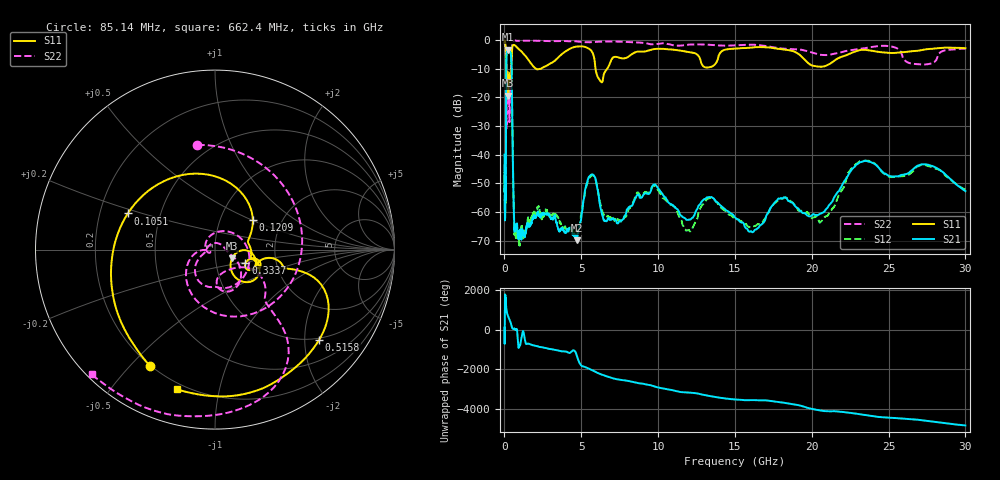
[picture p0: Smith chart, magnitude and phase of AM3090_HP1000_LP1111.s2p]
! Date/Time: Thu, Feb 28, 2019 2:02 PM
! Network Analyzer: Agilent Technologies E8364B Rev: A.07.50.67
! Sweep from 0.010 to 30.000 GHz, 1601 Points, Sweep Type: LOG
! Power Supply: 5.023 V, 0.002 A
# Hz S DB R 50
!freq MagS11 AngS11 MagS21 AngS21 MagS12 AngS12 MagS22 AngS22
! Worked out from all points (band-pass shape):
!   1601 points, 10 MHz to 30 GHz, reference 50 ohm
!   highest |S21| = -3.47 dB at 243.5 MHz (marker M1); lowest = -69.7 dB at 4.71 GHz (marker M2)
!   |S21| within 3 dB of the highest: 124.4 MHz to 442.2 MHz (317.7 MHz wide, 112 % of centre)
!   lowest |S11| = -19.5 dB at 243.5 MHz (marker M3), VSWR 1.24, Z = 60.2 - j5.77 ohm
!   |S11| at or under -10 dB: 118.4 MHz to 427.5 MHz (309 MHz wide, 113 % of centre); 2.035 GHz to 2.39 GHz (355.1 MHz wide, 16 % of centre); 5.925 GHz to 6.694 GHz (769.8 MHz wide, 12.2 % of centre)
!   |S22| runs from -30.8 to -0.2 dB; largest |S21 - S12| = 0.012
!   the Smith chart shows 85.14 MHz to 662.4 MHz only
!   S11 on the Smith chart (normalised r, x): 85.14 MHz: 0.20, -0.57; 105.1 MHz: 0.32, +0.18; 120.9 MHz: 1.43, +0.51; 333.7 MHz: 1.39, -0.22; 515.8 MHz: 0.96, -2.35; 662.4 MHz: 0.17, -0.75
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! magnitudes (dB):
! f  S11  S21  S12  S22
! 10 MHz  -0.3  -40.0  -43.4  -0.7
! 38.04 MHz  -0.5  -58.9  -57.9  -1.7
! 85.14 MHz  -2.6  -55.4  -52.9  -4.6
! 105.1 MHz  -5.6  -24.9  -25.0  -6.6
! 120.9 MHz  -11.4  -7.9  -7.9  -15.7
! 144.7 MHz  -13.8  -4.3  -4.3  -25.1
! 243.5 MHz  -19.5  -3.5  -3.4  -13.6
! 333.7 MHz  -14.6  -3.6  -3.6  -26.1
! 450.6 MHz  -8.0  -7.2  -7.2  -8.1
! 515.8 MHz  -2.3  -30.9  -30.7  -1.0
! 550.5 MHz  -1.9  -43.8  -43.5  -0.5
! 662.4 MHz  -1.9  -66.1  -67.7  -0.2
! 2.084 GHz  -10.2  -61.4  -59.7  -0.3
! 4.71 GHz  -2.3  -69.7  -67.5  -0.6
! 5.64 GHz  -3.7  -47.0  -47.5  -0.8
! 6.586 GHz  -10.8  -63.0  -61.0  -0.6
! 7.926 GHz  -6.3  -60.3  -61.5  -0.7
! 9.878 GHz  -3.1  -50.8  -51.2  -1.5
! 16.21 GHz  -2.6  -66.8  -64.9  -1.7
! 20.72 GHz  -9.3  -60.2  -62.7  -5.3
! 23.36 GHz  -3.5  -42.3  -42.2  -3.0
! 30 GHz  -2.9  -52.7  -52.1  -3.1
